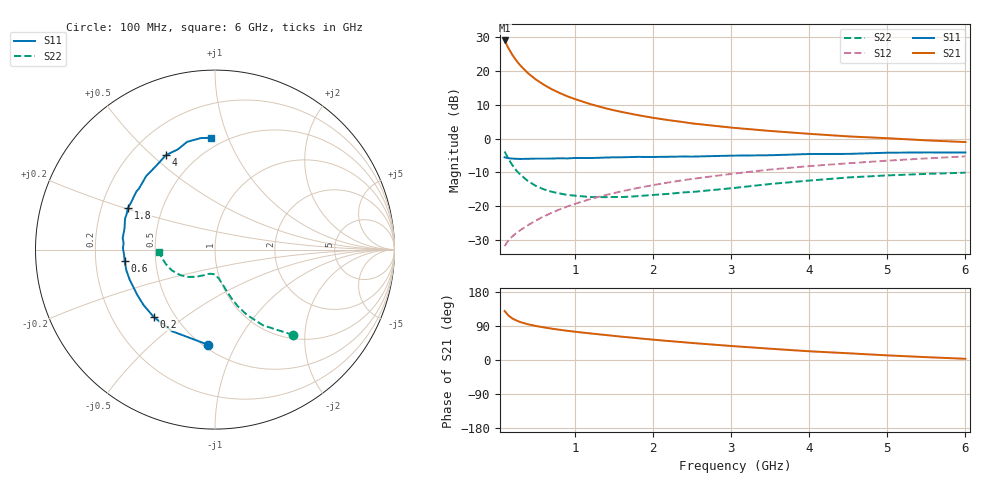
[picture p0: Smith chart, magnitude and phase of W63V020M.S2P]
! SIEMENS Small Signal Semiconductors
! BFR193W
! Si NPN RF Bipolar Junction Transistor in SOT323
! VCE = 3 V  IC = 20 mA
! Common Emitter S-Parameters:  September  1992
# GHz  S  MA  R  50
!  f  S11  S21  S12  S22
! GHz  MAG  ANG  MAG  ANG  MAG  ANG  MAG  ANG
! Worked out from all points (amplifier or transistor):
!   28 points, 100 MHz to 6 GHz, reference 50 ohm
!   highest |S21| = 29.1 dB at 100 MHz (marker M1)
!   |S21| within 3 dB of that: start of sweep to 167.2 MHz
!   unconditionally stable (mu >= 1): 746.4 MHz to 2.566 GHz
!   at 300 MHz: K = 0.76, MSG = 24.4 dB, |S12| = -27.1 dB
!   at 1.5 GHz: K = 1.04, MAG = 11.1 dB, |S12| = -16.1 dB
!   at 6 GHz: K = 0.91, MSG = 2.1 dB, |S12| = -5.2 dB
!   lowest NFmin = 1.40 dB at 450 MHz
!   S11 on the Smith chart (normalised r, x): 100 MHz: 0.53, -0.78; 200 MHz: 0.38, -0.39; 600 MHz: 0.33, -0.06; 1.8 GHz: 0.31, +0.21; 4 GHz: 0.34, +0.55; 6 GHz: 0.43, +0.87
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0.1  0.5306 -94.5  28.38 129.3  0.0257 58.2  0.6459 -47.5
0.15  0.5141 -117.8  21.71 117.3  0.0316 55.1  0.4997 -57.6
0.2  0.5075 -132.3  17.33 109.5  0.0358 54.8  0.4056 -63.9
0.25  0.5038 -142.4  14.3 104.3  0.0403 56.1  0.3384 -68.2
0.3  0.5013 -149.9  12.15 100.2  0.0442 57.4  0.2951 -70.8
0.4  0.5041 -160.4  9.286 94.2  0.0526 60.3  0.2353 -74.7
0.5  0.5074 -167.0  7.513 89.8  0.0615 62.7  0.2002 -77.3
0.6  0.5073 -172.8  6.304 86.1  0.0708 64.5  0.1786 -80.2
0.7  0.5076 -177.1  5.412 82.8  0.08 65.7  0.1644 -82.1
0.8  0.5131 179.1  4.769 79.9  0.0895 66.5  0.1554 -84.5
0.9  0.5103 175.8  4.249 77.2  0.099 67.0  0.1473 -86.2
1  0.5185 172.9  3.854 74.6  0.1087 67.4  0.1436 -88.1
1.2  0.5174 167.1  3.24 70.1  0.128 67.3  0.1371 -93.1
1.5  0.5301 160.9  2.631 63.6  0.1566 66.8  0.1372 -99.6
1.8  0.5378 154.4  2.236 57.6  0.1862 65.6  0.1411 -105.6
2.2  0.5407 146.2  1.881 50.1  0.2249 63.4  0.1527 -112.2
3  0.5611 133.1  1.459 37.0  0.3011 57.8  0.1847 -125.0
3.5  0.5687 125.8  1.301 29.8  0.3494 53.8  0.2138 -134.6
4  0.593 117.5  1.18 23.0  0.3927 49.4  0.2399 -143.7
4.5  0.5956 110.3  1.081 17.8  0.4324 45.2  0.2671 -154.3
5.5  0.6264 97.3  0.945 7.5  0.5107 36.8  0.3015 -172.2
6  0.6234 92.0  0.891 3.2  0.5478 32.2  0.314 -177.8
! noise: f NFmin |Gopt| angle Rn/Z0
0.45  1.4  0.3  160  0.1
0.9  1.45  0.34  172  0.11
1.8  2.2  0.56  -148  0.2
